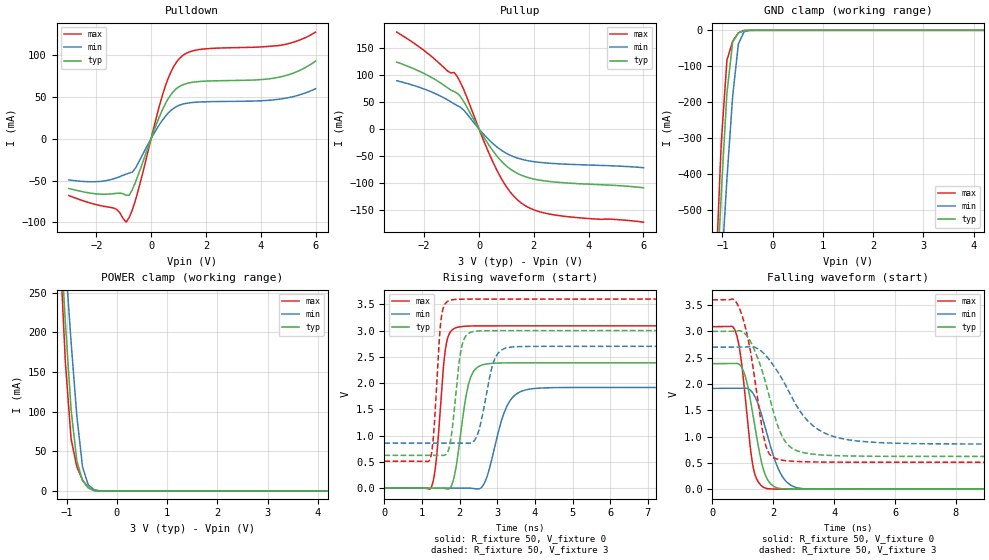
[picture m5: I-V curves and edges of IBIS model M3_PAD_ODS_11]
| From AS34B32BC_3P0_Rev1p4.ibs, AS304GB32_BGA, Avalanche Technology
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[Model] M3_PAD_ODS_11
Model_type I/O
Enable   Active-High
Vinl  =  0.8
Vinh  =  2.2
Vmeas =  1.5
Cref  =  30e-12
| Capacitance  typ   min   max
C_comp   6.128805e-12   5.681079e-12   6.591827e-12
| Variables   typ   min   max
[GND Clamp Reference]   0   0   0
[POWER Clamp Reference]   3   2.7   3.6
[Pulldown Reference]   0   0   0
[Pullup Reference]   3   2.7   3.6
[Temperature Range]   25   125   -40
[Voltage Range]   3   2.7   3.6
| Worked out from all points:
|   slope of the pulldown table from 0 to 0.45 V, typ, clamps not added: 12.2 ohm
|   slope of the pullup table from 0 to 0.45 V, typ, clamps not added: 12.3 ohm
|   GND clamp passes 1 mA (typ) near -0.57 V on its own axis
|   POWER clamp passes 1 mA (typ) near -0.47 V on its own axis
|   falling waveform, R_fixture 50, V_fixture 0: 20-80 % time 450ps typ, 615ps min, 341ps max; typ from 2.39 V to 0 V
|   falling waveform, R_fixture 50, V_fixture 3: 20-80 % time 750ps typ, 1.23ns min, 521ps max; typ from 3 V to 0.623 V
|   rising waveform, R_fixture 50, V_fixture 0: 20-80 % time 290ps typ, 443ps min, 201ps max; typ from 0 V to 2.39 V
|   rising waveform, R_fixture 50, V_fixture 3: 20-80 % time 213ps typ, 315ps min, 156ps max; typ from 0.623 V to 3 V
[GND Clamp]
| Voltage   I(typ)   I(min)   I(max)
-3V       -6.848A    -5.961A    -8.2A
-1.138V   -783.9mA   -953.3mA   -701.6mA
-1.024V   -456.3mA   -675.8mA   -315.2mA
-910.3mV  -174.6mA   -413.8mA   -83.06mA
-796.6mV  -33.06mA   -184.3mA   -30.65mA
-682.8mV  -7.332mA   -38.2mA    -7.06mA
-569mV    -713uA     -3.879mA   -286.8uA
-455.2mV  -15.31uA   -289.9uA   -1.608uA
6V        0A         0A         0A
[POWER Clamp]
| Voltage   I(typ)   I(min)   I(max)
-3V       2.695A     2.364A     3.234A
-1.138V   339.1mA    399.9mA    313.8mA
-1.024V   212.3mA    291.5mA    162.2mA
-910.3mV  102.5mA    187.9mA    65.61mA
-796.6mV  38.13mA    95.01mA    30.53mA
-682.8mV  12.94mA    30.26mA    13.87mA
-569mV    3.981mA    7.764mA    4.118mA
-455.2mV  618.9uA    1.561mA    450.1uA
-227.6mV  142.3nA    9.251uA    10.37nA
6V        0A         0A         0A
[Pulldown]
| Voltage   I(typ)   I(min)   I(max)
-3V       -59.47mA   -49.3mA    -67.99mA
-1.252V   -65.23mA   -46.75mA   -84.53mA
-910.3mV  -67.62mA   -42.31mA   -99.67mA
-796.6mV  -67.5mA    -41.16mA   -93.98mA
-569mV    -51.9mA    -35.1mA    -73.18mA
206.9mV   18.25mA    11.68mA    27.22mA
517.2mV   41.4mA     26.44mA    62.3mA
827.6mV   56.6mA     36.23mA    86.17mA
1.241V    65.21mA    41.79mA    100.9mA
1.966V    68.46mA    43.86mA    107mA
4.49V     72.13mA    46.26mA    110.5mA
6V        92.39mA    59.42mA    127mA
[Pullup]
| Voltage   I(typ)   I(min)   I(max)
-3V       124.2mA    89.58mA    180mA
-1.821V   98.19mA    70.66mA    138.4mA
-1.138V   76.16mA    53.74mA    107.4mA
-796.6mV  66.5mA     43.37mA    97.71mA
-569mV    51.88mA    35.59mA    74.49mA
103.4mV   -9.007mA   -6.076mA   -13.35mA
620.7mV   -48.21mA   -31.99mA   -73.47mA
1.034V    -70.25mA   -46.17mA   -109.9mA
1.552V    -86.01mA   -56.24mA   -137.9mA
2.069V    -93.69mA   -61.15mA   -151.5mA
2.793V    -98.65mA   -64.34mA   -160mA
6V        -109.3mA   -71.93mA   -173.1mA
[Ramp]
dV/dt_r   1.43201/0.290463n  1.14988/0.442819n  1.85402/0.201498n
dV/dt_f   1.42647/0.750331n  1.10595/1.2346n  1.85299/0.520805n
R_load = 50
[Falling Waveform]
R_fixture = 50
V_fixture = 0
V_fixture_min = 0
V_fixture_max = 0
| Time   V(typ)   V(min)   V(max)
0s        2.387V     1.916V     3.09V
768.5ps   2.391V     1.917V     2.983V
896.3ps   2.367V     1.917V     2.659V
1.035ns   2.226V     1.919V     2.011V
1.335ns   1.406V     1.822V     432.2mV
1.606ns   532.6mV    1.435V     69.33mV
1.816ns   178mV      1.004V     8.676mV
2.285ns   7.766mV    253mV      1.259mV
2.925ns   1.09mV     12.55mV    466uV
21.88ns   -1.114uV   701.6nV    -2.001uV
[Falling Waveform]
R_fixture = 50
V_fixture = 3
V_fixture_min = 2.7
V_fixture_max = 3.6
| Time   V(typ)   V(min)   V(max)
0s        3V         2.7V       3.6V
684.8ps   3.001V     2.7V       3.611V
919.3ps   3.011V     2.701V     3.395V
1.226ns   2.833V     2.712V     2.699V
1.721ns   2.084V     2.562V     905.3mV
2.171ns   1.168V     2.21V      564.8mV
2.557ns   803.1mV    1.806V     533.9mV
3.285ns   666.4mV    1.216V     517.6mV
4.744ns   628.4mV    916.9mV    512.4mV
21.88ns   622.5mV    856.8mV    511.7mV
[Rising Waveform]
R_fixture = 50
V_fixture = 0
V_fixture_min = 0
V_fixture_max = 0
| Time   V(typ)   V(min)   V(max)
0s        8.293nV    147.4nV    21.47nV
1.245ns   -252.2uV   -252uV     15.83mV
1.377ns   -278.9uV   -278.7uV   529.1mV
1.636ns   -13.69mV   -331.1uV   2.716V
1.945ns   590.1mV    -393.8uV   3.064V
2.28ns    2.087V     -1.337mV   3.087V
2.768ns   2.37V      312.8mV    3.09V
3.3ns     2.385V     1.62V      3.09V
4.012ns   2.386V     1.898V     3.09V
21.88ns   2.387V     1.916V     3.09V
[Rising Waveform]
R_fixture = 50
V_fixture = 3
V_fixture_min = 2.7
V_fixture_max = 3.6
| Time   V(typ)   V(min)   V(max)
0s        622.5mV    856.8mV    511.7mV
1.212ns   621.8mV    856.3mV    545.4mV
1.304ns   621.8mV    856.2mV    1.001V
1.518ns   621.6mV    856.1mV    3.276V
1.796ns   1.095V     856mV      3.586V
2.045ns   2.668V     855.9mV    3.598V
2.393ns   2.985V     907.6mV    3.599V
2.912ns   2.999V     2.422V     3.599V
3.375ns   2.999V     2.686V     3.599V
21.88ns   3V         2.7V       3.6V
